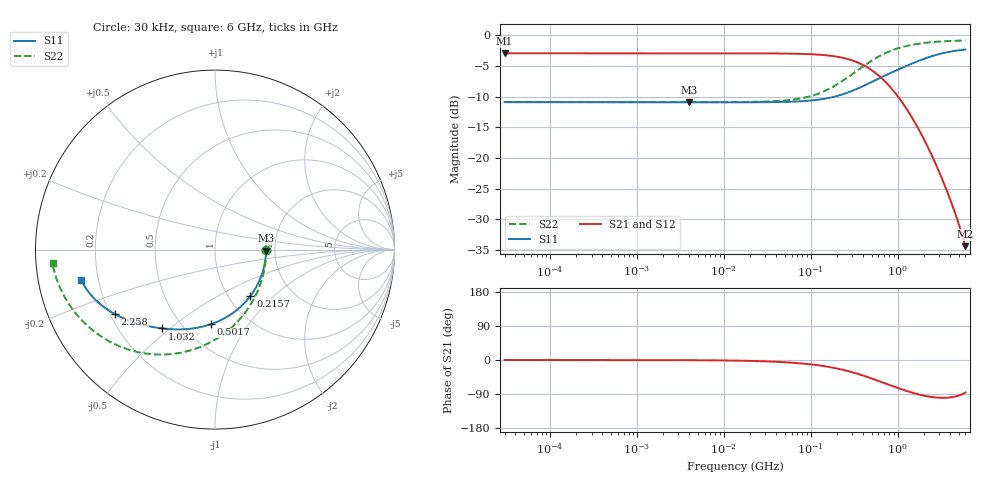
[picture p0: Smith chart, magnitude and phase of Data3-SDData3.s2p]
!EMIF06-MSD04F3
!Simulation
!24/03/11  09:28
!Start Freq. :30.000kHz; Stop Freq. : 6.000GHz
!Number of points : 1592; Sweep : LOGARITHMIC
!D1-D4 (Data3/CD-SDData3/CD)
!Freq ReS11 ImS11 ReS21 ImS21 ReS12 ImS12 ReS22 ImS22
# Hz  S  RI  R  50
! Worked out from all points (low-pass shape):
!   1592 points, 30 kHz to 6 GHz, reference 50 ohm
!   highest |S21| = -2.92 dB at 30 kHz (marker M1); lowest = -34.4 dB at 6 GHz (marker M2)
!   |S21| within 3 dB of the highest: start of sweep to 529.7 MHz
!   lowest |S11| = -10.9 dB at 3.955 MHz (marker M3), VSWR 1.79, Z = 89.7 - j1.05 ohm
!   |S11| at or under -10 dB: start of sweep to 187.4 MHz
!   |S22| runs from -10.9 to -0.8 dB; largest |S21 - S12| = 2.3e-15
!   S11 on the Smith chart (normalised r, x): 30 kHz: 1.80, -0.00; 215.7 MHz: 1.26, -0.73; 501.7 MHz: 0.68, -0.68; 1.032 GHz: 0.38, -0.47; 2.258 GHz: 0.22, -0.28; 6 GHz: 0.13, -0.11
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30000  0.2855 -0.000524  0.7142 -0.000312  0.7142 -0.000312  0.2857 -0.000211
231093.6  0.2844 -0.000816  0.7135 -0.000615  0.7135 -0.000615  0.2853 -0.000631
1766531  0.2841 -0.00251  0.7134 -0.00264  0.7134 -0.00264  0.2852 -0.00367
3954770  0.2841 -0.00539  0.7133 -0.00577  0.7133 -0.00577  0.2852 -0.00815
1.350376e7  0.2837 -0.0182  0.7129 -0.0196  0.7129 -0.0196  0.2846 -0.0277
4.336319e7  0.2801 -0.058  0.7084 -0.0624  0.7084 -0.0624  0.2785 -0.0885
6.820056e7  0.2743 -0.0905  0.7012 -0.0973  0.7012 -0.0973  0.2686 -0.1381
1.032257e8  0.2622 -0.1348  0.6859 -0.1444  0.6859 -0.1444  0.248 -0.2052
1.538584e8  0.2372 -0.1944  0.6547 -0.2067  0.6547 -0.2067  0.2056 -0.2944
2.156691e8  0.1975 -0.258  0.6054 -0.2707  0.6054 -0.2707  0.1385 -0.3871
3.239325e8  0.1145 -0.3422  0.5039 -0.3476  0.5039 -0.3476  -0.00042 -0.5021
4.078069e8  0.0474 -0.3854  0.4239 -0.3788  0.4239 -0.3788  -0.1105 -0.5531
5.017121e8  -0.0236 -0.4161  0.3419 -0.3914  0.3419 -0.3914  -0.2246 -0.5798
6.267888e8  -0.1071 -0.4369  0.2507 -0.3844  0.2507 -0.3844  -0.3536 -0.5826
7.890804e8  -0.1957 -0.4447  0.1629 -0.3546  0.1629 -0.3546  -0.4818 -0.5569
1.032257e9  -0.2962 -0.4391  0.0805 -0.2986  0.0805 -0.2986  -0.6106 -0.4988
1.492066e9  -0.4252 -0.4128  0.012 -0.2077  0.012 -0.2077  -0.7395 -0.3961
2.258333e9  -0.5562 -0.3601  -0.0133 -0.119  -0.0133 -0.119  -0.8276 -0.2814
2.9543e9  -0.6283 -0.3127  -0.013 -0.0777  -0.013 -0.0777  -0.8621 -0.2156
3.805876e9  -0.6829 -0.2617  -0.00811 -0.05  -0.00811 -0.05  -0.8837 -0.1607
4.64645e9  -0.7161 -0.22  -0.00364 -0.0342  -0.00364 -0.0342  -0.8952 -0.1218
6e9  -0.7473 -0.1678  0.00147 -0.0191  0.00147 -0.0191  -0.9049 -0.0766
